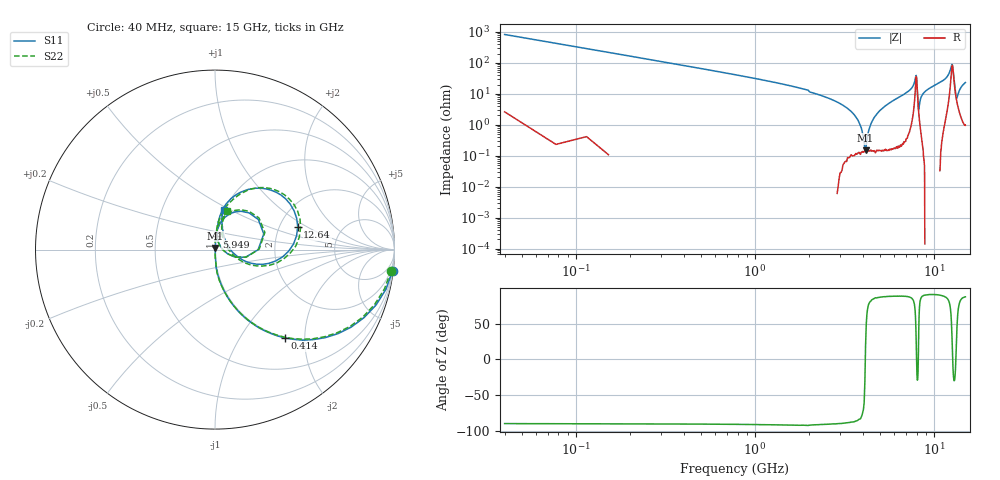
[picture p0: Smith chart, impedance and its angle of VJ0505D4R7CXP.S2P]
! VJ0505D4R7CXP
! MLCC placed on 25 mil thick microstrip substrate in series configuraton.
! DATE 06/29/2018  07:49
! CORRECTED  DATA
# GHz  S  MA  R  50.00
!  FREQ  S11M  S11A  S21M  S21A  S12M  S12A  S22M  S22A
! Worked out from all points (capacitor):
!   401 points, 40 MHz to 15 GHz, reference 50 ohm
!   read as one part in series: C = 4.79 pF near 114.8 MHz
!   lowest |Z| = 150 mohm at 4.154 GHz (marker M1)
!   series resonance near 4.141 GHz, so ESL is about 310 pH
!   S11 on the Smith chart (normalised r, x): 40 MHz: 1, -17; 414 MHz: 0.99, -1.60; 5.949 GHz: 1.00, +0.15; 12.64 GHz: 2.52, +0.83; 15 GHz: 1.00, +0.46
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0.04  0.9962 -6.8  0.1202 83.0  0.1201 83.3  0.9886 -6.8
0.1896  0.8722 -29.8  0.4964 60.5  0.4968 60.4  0.8649 -29.7
0.414  0.6272 -51.7  0.7853 38.8  0.7857 38.8  0.6219 -51.6
1.0124  0.2972 -73.7  0.961 17.5  0.9615 17.5  0.2956 -73.8
2.5458  0.06822 -86.6  0.9977 4.6  0.9982 4.6  0.06815 -86.8
3.5182  0.01546 -83.8  0.998 1.8  0.9987 1.8  0.01528 -88.9
3.7052  0.007847 -77.4  0.9981 1.4  0.9984 1.4  0.007555 -92.0
3.8922  0.00201 -8.7  0.9982 1.0  0.9988 1.0  0.0006155 -153.7
4.154  0.009916 78.1  0.9978 0.5  0.9984 0.5  0.01006 91.8
5.0516  0.04152 85.6  0.997 -1.2  0.9974 -1.1  0.04096 89.4
5.9492  0.07365 85.1  0.995 -2.8  0.9956 -2.8  0.07281 87.2
7.52  0.1607 77.5  0.9746 -7.9  0.9753 -7.9  0.1639 78.9
7.9314  0.294 34.8  0.7708 -11.1  0.7718 -11.1  0.3019 35.9
8.2306  0.03889 50.5  0.9751 -0.4  0.9755 -0.4  0.03753 52.7
8.6794  0.1072 83.5  0.9912 -5.0  0.992 -5.0  0.1101 85.3
10.0258  0.1894 81.7  0.9826 -9.8  0.984 -9.8  0.1943 80.3
11.821  0.3238 69.3  0.92 -18.3  0.9207 -18.3  0.3351 66.2
12.5316  0.4897 31.1  0.6179 -22.5  0.6186 -22.6  0.5067 29.6
12.6438  0.478 15.4  0.5425 -11.5  0.543 -11.5  0.4911 14.1
12.9056  0.2757 -17.4  0.7433 7.8  0.7437 7.8  0.2793 -19.2
13.3544  0.07305 23.2  0.9354 -1.0  0.9362 -1.0  0.06525 25.0
15  0.2249 77.4  0.964 -12.8  0.9644 -12.8  0.2249 72.6
